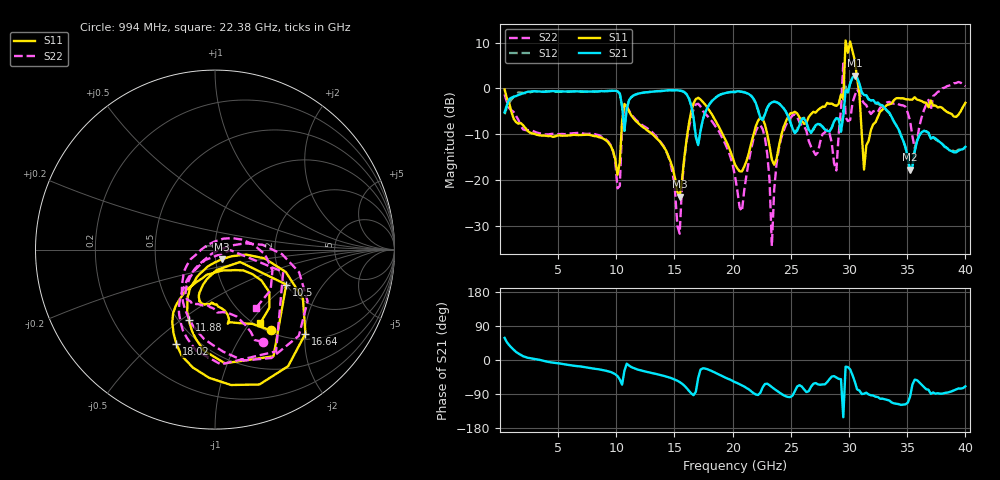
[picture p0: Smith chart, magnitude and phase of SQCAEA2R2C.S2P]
! Network Analyzer HP8722ES.07.66: Jul 25, 2000 Serial No. US39175408
! 26 Oct 2004  12:54:23
! Frequency  S11  S21  S12  S22
# HZ  S  DB R  50
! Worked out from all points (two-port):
!   201 points, 400 MHz to 40 GHz, reference 50 ohm
!   highest |S21| = 2.78 dB at 30.5 GHz (marker M1); lowest = -17.8 dB at 35.25 GHz (marker M2)
!   |S21| within 3 dB of the highest: 29.97 GHz to 31.03 GHz (1.061 GHz wide, 3.48 % of centre)
!   lowest |S11| = -23.7 dB at 15.45 GHz (marker M3), VSWR 1.14, Z = 53.5 - j5.83 ohm
!   |S11| at or under -10 dB: 3.04 GHz to 10.43 GHz (7.394 GHz wide, 110 % of centre); 13.1 GHz to 16.1 GHz (3.003 GHz wide, 20.6 % of centre); 19.13 GHz to 21.8 GHz (2.665 GHz wide, 13 % of centre)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
!   |S22| runs from -34.5 to 5.5 dB; largest |S21 - S12| = 0.25
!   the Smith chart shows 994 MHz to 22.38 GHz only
!   S11 on the Smith chart (normalised r, x): 994 MHz: 1.03, -1.33; 10.5 GHz: 2.00, -0.97; 11.88 GHz: 0.56, -0.54; 16.64 GHz: 1.13, -2.01; 18.02 GHz: 0.39, -0.60; 22.38 GHz: 1.06, -1.13
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4e8  -0.23 -33.2  -5.17 58.3  -5.63 63.6  -1.29 -24.6
9.94e8  -5.22 -55.3  -1.98 32.5  -2.38 29.4  -4.76 -62.6
7.132e9  -10.15 -103.3  -0.66 -18.1  -0.71 -18.6  -9.84 -114.2
1.0498e10  -7.09 -26.2  -3.82 -65.1  -4.08 -66.3  -7.97 -18.1
1.1884e10  -7.57 -110.3  -1.13 -25.8  -1.12 -25.6  -7.30 -116.9
1.3666e10  -11.36 -121.9  -0.60 -38.8  -0.56 -38.6  -11.25 -129.5
1.5448e10  -23.68 -55.9  -0.49 -58.2  -0.43 -58.7  -31.73 -0.1
1.6636e10  -3.25 -42.9  -6.36 -92.9  -6.49 -93.1  -4.57 -29.1
1.8022e10  -4.91 -112.2  -3.37 -26.7  -3.36 -26.6  -6.58 -101.8
2.02e10  -16.61 -108.4  -0.80 -58.6  -0.65 -57.9  -19.17 -164.9
2.2378e10  -6.35 -58.4  -6.44 -86.6  -6.54 -85.4  -8.01 -55.3
2.3368e10  -15.55 -78.9  -3.03 -71.4  -2.99 -71.2  -34.47 148.0
2.6932e10  -5.10 -46.7  -8.80 -62.8  -9.05 -63.1  -13.62 -45.2
2.8912e10  -3.80 -36.0  -6.50 -46.1  -6.49 -45.4  -17.91 23.5
2.9506e10  -2.34 6.6  -6.13 -151.1  -5.07 -131.2  5.46 37.8
2.9704e10  10.50 0.8  -0.41 -17.8  0.43 -4.7  -6.29 -51.5
3.01e10  10.29 -73.4  1.07 -25.0  1.19 -25.3  -6.87 19.0
3.0496e10  6.17 -102.8  2.78 -56.8  2.75 -55.9  -1.54 -9.1
3.0694e10  2.16 45.9  2.35 -77.6  2.16 -77.1  -0.19 152.7
3.3466e10  -3.47 -23.7  -5.29 -106.8  -5.41 -106.4  -2.93 -37.3
3.5248e10  -2.42 -45.9  -17.77 -96.6  -18.15 -92.6  -7.04 -95.1
4e10  -3.15 -38.7  -12.74 -69.4  -12.71 -68.4  0.52 -6.8
